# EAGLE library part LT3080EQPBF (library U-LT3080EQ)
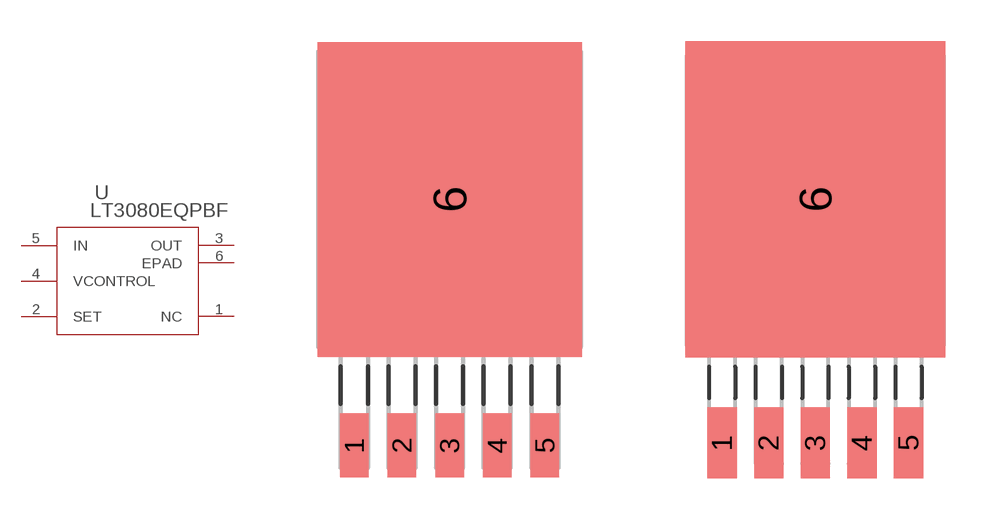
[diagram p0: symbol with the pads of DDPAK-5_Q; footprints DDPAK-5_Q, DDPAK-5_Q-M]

Designator prefix U

## LT3080EQPBF (MANUFACTURER_PART_NUMBER: LT3080EQ#PBF; VENDOR: Linear Technology)  [DDPAK-5_Q]
1  NC  nc
2  SET  in
3  OUT  pwr
4  VCONTROL  in
5  IN  pwr
6  EPAD  pwr

## LT3080EQPBFDDPAK-5_Q-M (MANUFACTURER_PART_NUMBER: LT3080EQ#PBF; VENDOR: Linear Technology)  [DDPAK-5_Q-M]
Pads as for DDPAK-5_Q

## LT3080EQPBFDDPAK-5_Q-L (MANUFACTURER_PART_NUMBER: LT3080EQ#PBF; VENDOR: Linear Technology)  [DDPAK-5_Q-L]
Pads as for DDPAK-5_Q

## Footprint DDPAK-5_Q (pad centres in mm)
smd 1.016 x 2.286: 1 -3.404,-8.801; 2 -1.702,-8.801; 3 0,-8.801; 4 1.702,-8.801; 5 3.404,-8.801
smd 9.449 x 11.252: 6 0,0

## Footprint DDPAK-5_Q-M (pad centres in mm)
smd 1.067 x 2.591: 1 -3.404,-8.852; 2 -1.702,-8.852; 3 0,-8.852; 4 1.702,-8.852; 5 3.404,-8.852
smd 9.5 x 11.557: 6 0,0.051

## Footprint DDPAK-5_Q-L (pad centres in mm)
smd 0.965 x 1.981: 1 -3.404,-8.75; 2 -1.702,-8.75; 3 0,-8.75; 4 1.702,-8.75; 5 3.404,-8.75
smd 9.398 x 10.947: 6 0,-0.051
